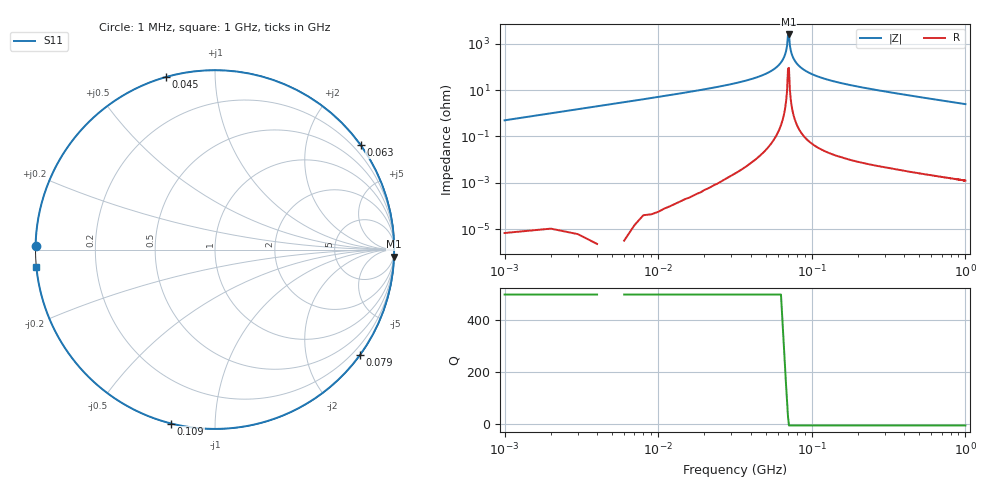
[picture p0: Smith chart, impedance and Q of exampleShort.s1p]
# MHz S RI R 50.0
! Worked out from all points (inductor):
!   999 points, 1 MHz to 1 GHz, reference 50 ohm
!   read as one part to ground: L = 79.1 nH near 5 MHz
!   highest |Z| = 2.51 kohm at 71 MHz (marker M1)
!   self-resonance near 70 MHz
!   S11 on the Smith chart (normalised r, x): 1 MHz: 0.00, +0.01; 45 MHz: 0.00, +0.75; 63 MHz: 0.01, +3.11; 79 MHz: 0.01, -3.07; 109 MHz: 0.00, -0.78; 1 GHz: 0.00, -0.05
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1  -0.9998 0.0199
15  -0.9524 0.3049
27  -0.8199 0.5724
37  -0.5901 0.8071
45  -0.274 0.9614
50  -6.9e-05 0.9995
55  0.3219 0.946
59  0.5853 0.8097
63  0.8113 0.5826
67  0.9572 0.2848
71  0.9978 -0.0397
75  0.9383 -0.3417
79  0.8075 -0.5874
85  0.5522 -0.8321
91  0.2969 -0.9536
100  -0.0174 -0.9989
109  -0.2438 -0.969
126  -0.5079 -0.8607
145  -0.6674 -0.744
170  -0.7802 -0.6249
204  -0.859 -0.5114
251  -0.9124 -0.4087
376  -0.9634 -0.2674
502  -0.9799 -0.1988
626  -0.9872 -0.1589
751  -0.9912 -0.1322
876  -0.9935 -0.1132
1000  -0.995 -0.0991
